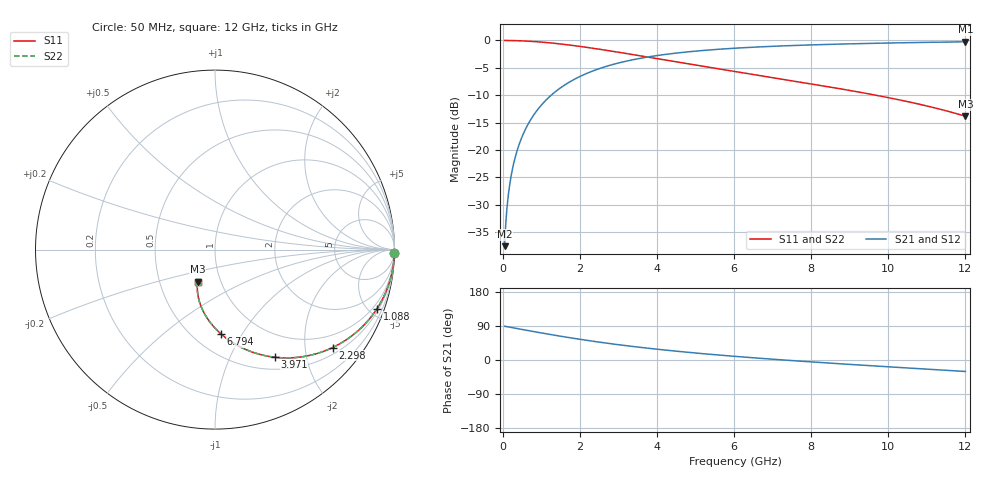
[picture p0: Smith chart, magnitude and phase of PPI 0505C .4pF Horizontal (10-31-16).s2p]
# MHz S MA R 50
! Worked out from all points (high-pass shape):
!   1601 points, 50 MHz to 12 GHz, reference 50 ohm
!   highest |S21| = -0.25 dB at 12 GHz (marker M1); lowest = -37.5 dB at 50 MHz (marker M2)
!   |S21| within 3 dB of the highest: 3.576 GHz to end of sweep
!   lowest |S11| = -13.8 dB at 12 GHz (marker M3), VSWR 1.51, Z = 38.8 - j14.5 ohm
!   |S11| at or under -10 dB: 9.682 GHz to end of sweep
!   |S22| runs from -13.8 to 0.0 dB; largest |S21 - S12| = 0
!   S11 on the Smith chart (normalised r, x): 50 MHz: open; 1.088 GHz: 0.65, -5.57; 2.298 GHz: 0.65, -2.62; 3.971 GHz: 0.66, -1.49; 6.794 GHz: 0.67, -0.81; 12 GHz: 0.78, -0.29
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50  0.9999 -0.9  0.01326 89.1  0.01326 89.1  0.9999 -0.9
79.875  0.9998 -1.5  0.02119 88.5  0.02119 88.5  0.9998 -1.5
139.625  0.9993 -2.6  0.03702 87.4  0.03702 87.4  0.9993 -2.6
191.9062  0.9987 -3.6  0.05084 86.4  0.05084 86.4  0.9987 -3.6
274.0625  0.9973 -5.2  0.07251 84.8  0.07251 84.8  0.9973 -5.2
371.1562  0.9951 -7.0  0.09799 83.0  0.09799 83.0  0.9951 -7.0
505.5938  0.9911 -9.5  0.1329 80.5  0.1329 80.5  0.9911 -9.5
669.9062  0.9845 -12.5  0.175 77.4  0.175 77.4  0.9845 -12.5
864.0938  0.9746 -16.1  0.2234 73.9  0.2234 73.9  0.9746 -16.1
1088.156  0.9605 -20.1  0.2773 69.9  0.2773 69.9  0.9605 -20.1
1521.344  0.9269 -27.6  0.3741 62.4  0.3741 62.4  0.9269 -27.6
2044.156  0.8784 -36.0  0.4765 54.0  0.4765 54.0  0.8784 -36.0
2298.094  0.853 -39.8  0.5203 50.1  0.5203 50.1  0.853 -39.8
3059.906  0.7749 -50.2  0.6299 39.6  0.6299 39.6  0.7749 -50.2
3971.094  0.6857 -61.0  0.7251 28.8  0.7251 28.8  0.6857 -61.0
4038.312  0.6794 -61.7  0.7309 28.1  0.7309 28.1  0.6794 -61.7
4994.312  0.5971 -71.2  0.7988 18.5  0.7988 18.5  0.5971 -71.2
6025  0.5208 -80.0  0.8498 9.6  0.8498 9.6  0.5208 -80.0
6794.281  0.4709 -85.9  0.8779 3.6  0.8779 3.6  0.4709 -85.9
8019.156  0.4007 -94.5  0.9113 -5.1  0.9113 -5.1  0.4007 -94.5
10013.31  0.3002 -107.0  0.9479 -18.0  0.9479 -18.0  0.3002 -107.0
12000  0.2034 -118.4  0.9718 -30.3  0.9718 -30.3  0.2034 -118.4
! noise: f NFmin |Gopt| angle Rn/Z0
50  0.002254  0.9868  0.902  0.03918
1372  0.005974  0.7938  9.801  0.00594
2701  0.009087  0.7263  14.24  0.006501
4031  0.01189  0.6895  18.56  0.007259
5360  0.01454  0.666  22.87  0.008034
6682  0.0171  0.6507  27.11  0.008816
8012  0.01967  0.641  31.3  0.009633
9341  0.02228  0.6356  35.4  0.0105
1.067e+04  0.02497  0.6338  39.39  0.01144
1.2e+04  0.02778  0.635  43.27  0.01248
